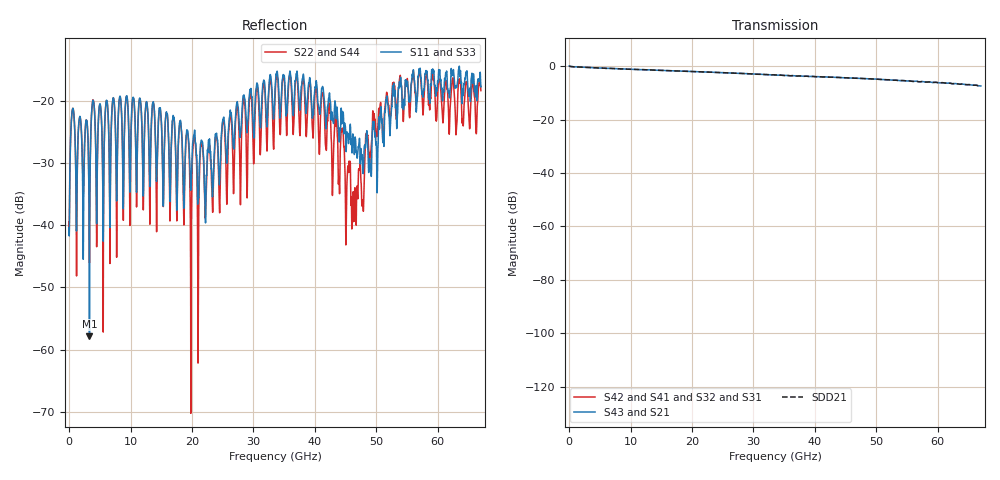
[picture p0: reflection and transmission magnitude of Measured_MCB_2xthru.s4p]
# GHz S RI R 50
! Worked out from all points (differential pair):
!   6700 points, 10 MHz to 67 GHz, reference 50 ohm
!   strongest paths, dB at 10 MHz, 16.76 GHz, 33.51 GHz, 50.26 GHz, 67 GHz:
!     S43: 0.0, -1.7, -3.3, -4.9, -7.4
!     S21: 0.0, -1.7, -3.3, -4.9, -7.4
!     S42: -, -, -, -, -
!     S41: -, -, -, -, -
!     S32: -, -, -, -, -
!     S31: -, -, -, -, -
!   taken as a pair (ports 3,1 in; 4,2 out), SDD21 dB: 0.0, -1.7, -3.3, -4.9, -7.4
!   lowest |S11| = -57.9 dB at 3.32 GHz (marker M1), VSWR 1.00, Z = 49.9 + j0.0429 ohm
!   |S11| at or under -10 dB: start of sweep to end of sweep
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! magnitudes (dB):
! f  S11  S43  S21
! 10 MHz  -40.4  0.0  0.0
! 3.32 GHz  -57.9  -0.5  -0.5
! 21.02 GHz  -35.5  -2.1  -2.1
! 35.93 GHz  -15.3  -3.6  -3.6
! 46.15 GHz  -25.4  -4.4  -4.4
! 52.75 GHz  -18.0  -5.3  -5.3
! 67 GHz  -17.8  -7.4  -7.4
